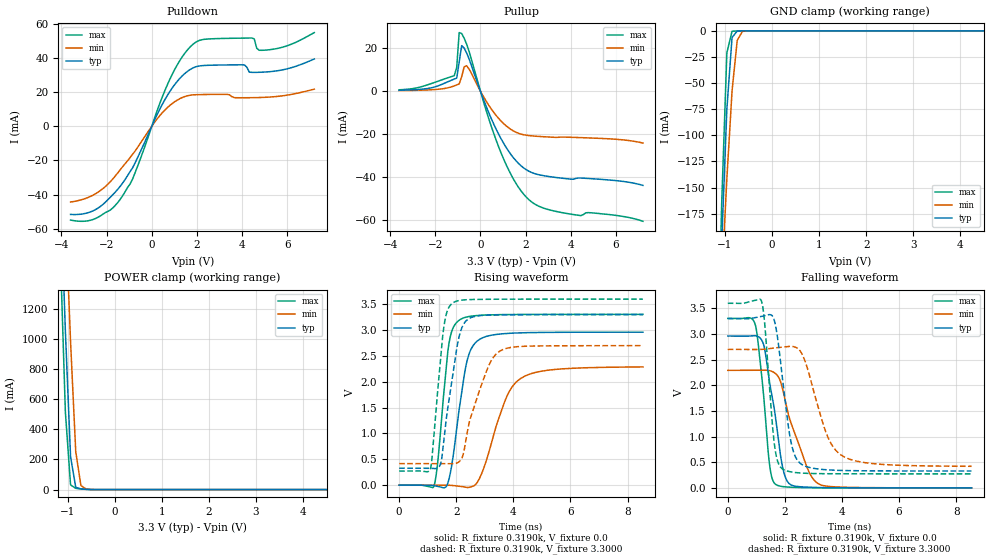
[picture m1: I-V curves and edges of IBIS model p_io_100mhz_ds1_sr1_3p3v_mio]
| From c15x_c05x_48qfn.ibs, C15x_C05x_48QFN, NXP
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[Model] p_io_100mhz_ds1_sr1_3p3v_mio
|   Model p_io_100mhz_ds1_sr1_3p3v_mio
| This model was characterised for following simulation conditions:
| External (pad) voltage:
|   - Typ: 3.3V,   - Min: 2.7V,   - Max: 3.6V
| Library cells for typ/min/max conditions are connected as defined below:
|  pad - External Pad
|  ipp_do_lv - Core Input
|  ipp_obe_lv - Output Buffer Enable
|  IOGC - NC
|  REFH3V3 - REFH3V3
|  REFL3V3 - REFL3V3
|  ZI - NC
|  abut_ncal_vddio[1] - vddio
|  abut_ncal_vddio[2] - vddio
|  abut_ncal_vddio[3] - vssio
|  abut_ncal_vddio[4] - vddio
|  abut_ncal_vddio[5] - vddio
|  abut_ncal_vddio[6] - vssio
|  abut_pcal_vddio[1] - vssio
|  abut_pcal_vddio[2] - vssio
|  abut_pcal_vddio[3] - vddio
|  abut_pcal_vddio[4] - vssio
|  abut_pcal_vddio[5] - vssio
|  abut_pcal_vddio[6] - vddio
|  ipp_do_1p8v - ipp_do_1p8v
|  ipp_dse_lv - vdd_lv
|  ipp_eftd_lv - NC
|  ipp_ina_mux_vddio - NC
|  ipp_ina_mux_vddio[0] - NC
|  ipp_ina_mux_vddio[1] - NC
|  ipp_ina_r0_vddio - NC
|  ipp_ina_r0a_vddio - NC
|  ipp_ina_r0b_vddio - NC
|  ipp_ina_r0c_vddio - NC
|  ipp_ina_r0d_vddio - NC
|  ipp_ina_r0e_vddio - NC
|  ipp_ina_r0f_vddio - NC
|  ipp_ina_r300_vddio - NC
|  ipp_ina_r300a_vddio - NC
|  ipp_ina_r300b_vddio - NC
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Model_type I/O
Polarity   Non-Inverting
Enable   Active-High
Vinl =   0.9900V
Vinh =   2.3100V
Vmeas =  1.6500V
Cref =   30.0000pF
Rref =   1.0000M
Vref =   3.3000V
C_comp   1.3234pF   1.2639pF   1.4076pF
|C_comp_pullup   0.6740pF   0.7057pF   0.6520pF
|C_comp_pulldown   0.5815pF   0.6343pF   0.5433pF
[Model Spec]
| variable   typ   min   max
Vinh   2.3100V   1.8900V   2.5200V
Vinl   0.9900V   0.8100V   1.0800V
[Temperature Range]   25.0000   0.1250k   -40.0000
[Voltage Range]   3.3000V   2.7000V   3.6000V
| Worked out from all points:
|   slope of the pulldown table from 0 to 0.495 V, typ, clamps not added: 36.6 ohm
|   slope of the pullup table from 0 to 0.495 V, typ, clamps not added: 37.7 ohm
|   GND clamp passes 1 mA (typ) near -0.75 V on its own axis
|   POWER clamp passes 1 mA (typ) near -0.55 V on its own axis
|   rising waveform, R_fixture 0.3190k, V_fixture 0.0: 20-80 % time 463ps typ, 832ps min, 328ps max; typ from 0 V to 2.96 V
|   rising waveform, R_fixture 0.3190k, V_fixture 3.3000: 20-80 % time 462ps typ, 748ps min, 321ps max; typ from 0.328 V to 3.3 V
|   falling waveform, R_fixture 0.3190k, V_fixture 0.0: 20-80 % time 473ps typ, 774ps min, 322ps max; typ from 2.96 V to 0 V
|   falling waveform, R_fixture 0.3190k, V_fixture 3.3000: 20-80 % time 407ps typ, 769ps min, 280ps max; typ from 3.3 V to 0.329 V
[Pulldown]
|Voltage   I(typ)   I(min)   I(max)
-3.6V     -51.52mA   -44.27mA   -54.81mA
-2.5V     -48.75mA   -39.51mA   -53.96mA
-1.4V     -35.12mA   -25.45mA   -42.73mA
-850mV    -24.27mA   -16.41mA   -30.84mA
800mV     20.29mA    12.16mA    27.43mA
1.35V     29.44mA    16.78mA    40.57mA
1.9V      34.5mA     18.39mA    48.67mA
4.1V      35.87mA    16.66mA    51.51mA
4.43V     31.5mA     16.69mA    51.59mA
4.65V     31.5mA     16.75mA    45.53mA
5.09V     31.75mA    16.96mA    44.55mA
7.2V      39.3mA     21.67mA    54.74mA
[Pullup]
|Voltage   I(typ)   I(min)   I(max)
-3.6V     391.8uA    234.9uA    605.7uA
-1.16V    5.604mA    2.419mA    7.14mA
-1.05V    6.055mA    2.871mA    11mA
-940mV    13.56mA    3.339mA    27.24mA
-830mV    21.15mA    6.685mA    26.82mA
-720mV    20.05mA    11.26mA    24.61mA
-610mV    17.74mA    11.81mA    21.86mA
820mV     -20.29mA   -12.86mA   -26.23mA
1.48V     -31.23mA   -18.63mA   -41.23mA
2.03V     -36.57mA   -20.53mA   -49.31mA
3.46V     -40.33mA   -21.49mA   -56.22mA
7.2V      -43.87mA   -24.17mA   -60.58mA
[GND_clamp]
|Voltage   I(typ)   I(min)   I(max)
-3.6V     -4.134A    -3.035A    -5.609A
-1.18V    -349.4mA   -343.6mA   -365.7mA
-1.07V    -202.9mA   -239.3mA   -165.2mA
-960mV    -74.83mA   -141.5mA   -21.03mA
-850mV    -6.389mA   -57.64mA   -383.3uA
-740mV    -222.1uA   -9.174mA   -124.1uA
-630mV    -55.93uA   -558.9uA   -58.07uA
7.2V      0A         0A         0A
[POWER_clamp]
|Voltage   I(typ)   I(min)   I(max)
-3.6V     24.54A     22.33A     26.93A
-1.16V    2.046A     2.721A     1.599A
-1.05V    1.052A     1.847A     514.4mA
-940mV    218.6mA    981.8mA    31.16mA
-830mV    15.1mA     252.4mA    8.462mA
-720mV    4.281mA    26.81mA    4.453mA
-610mV    1.717mA    3.626mA    1.66mA
7.2V      0A         0A         0A
[Ramp]
| variable   typ   min   max
dV/dt_r  1.7762/0.4627n   1.3728/0.8323n   1.9832/0.3278n
dV/dt_f  1.7828/0.4074n   1.3676/0.7690n   1.9962/0.2798n
R_load = 0.3190k
[Rising Waveform]
R_fixture= 0.3190k
V_fixture= 0.0
V_fixture_min= 0.0
V_fixture_max= 0.0
|time   V(typ)   V(min)   V(max)
0s        2.902nV    250nV      9.459nV
1.223ns   -10.89mV   -6.469uV   -14.68mV
1.367ns   -23.26mV   432.8uV    521.7mV
1.741ns   105.6mV    -943.7uV   2.727V
2.104ns   1.469V     -19.16mV   3.193V
2.362ns   2.366V     -44.86mV   3.254V
2.644ns   2.739V     -3.7mV     3.278V
3.78ns    2.936V     1.726V     3.302V
4.288ns   2.948V     2.075V     3.304V
8.54ns    2.96V      2.288V     3.305V
[Rising Waveform]
R_fixture= 0.3190k
V_fixture= 3.3000
V_fixture_min= 2.7000
V_fixture_max= 3.6000
|time   V(typ)   V(min)   V(max)
0s        328.4mV    417.4mV    273mV
1.095ns   327.1mV    417.3mV    314.6mV
1.431ns   382.4mV    418mV      2.336V
1.553ns   812.4mV    418.4mV    3.011V
1.88ns    2.147V     415.2mV    3.527V
2.089ns   2.846V     449mV      3.572V
2.297ns   3.149V     734.8mV    3.587V
2.949ns   3.286V     2.042V     3.597V
3.527ns   3.295V     2.594V     3.599V
8.54ns    3.3V       2.7V       3.6V
[Falling Waveform]
R_fixture= 0.3190k
V_fixture= 0.0
V_fixture_min= 0.0
V_fixture_max= 0.0
|time   V(typ)   V(min)   V(max)
0s        2.961V     2.292V     3.305V
969.3ps   2.966V     2.29V      3.171V
1.26ns    2.783V     2.295V     1.777V
1.471ns   2.038V     2.285V     420.1mV
1.688ns   1.313V     2.221V     63.57mV
1.9ns     459.6mV    1.975V     27.02mV
2.078ns   134.8mV    1.527V     16.67mV
2.798ns   12.69mV    370.4mV    3.524mV
3.163ns   6.584mV    83.26mV    1.82mV
8.54ns    86.29uV    287.2uV    52.59uV
[Falling Waveform]
R_fixture= 0.3190k
V_fixture= 3.3000
V_fixture_min= 2.7000
V_fixture_max= 3.6000
|time   V(typ)   V(min)   V(max)
0s        3.3V       2.7V       3.6V
1.18ns    3.345V     2.7V       3.643V
1.299ns   3.357V     2.705V     3.175V
1.639ns   3.248V     2.728V     824.4mV
1.919ns   2.115V     2.746V     368.1mV
2.245ns   816.2mV    2.759V     308.4mV
2.666ns   434.4mV    2.531V     285.8mV
3.46ns    352.5mV    1.052V     275.7mV
4ns       339.2mV    629.7mV    274.2mV
8.54ns    328.6mV    420.6mV    273.1mV
